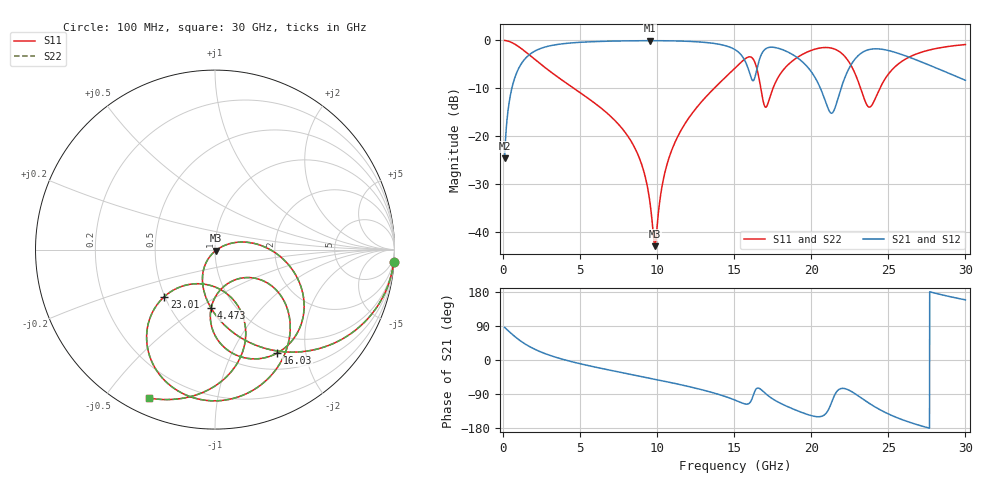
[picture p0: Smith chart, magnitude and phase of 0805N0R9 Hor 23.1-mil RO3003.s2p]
# GHz S MA R 50
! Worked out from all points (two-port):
!   3201 points, 100 MHz to 30 GHz, reference 50 ohm
!   highest |S21| = -0.06 dB at 9.556 GHz (marker M1); lowest = -24.7 dB at 100 MHz (marker M2)
!   |S21| within 3 dB of the highest: 1.679 GHz to 15.46 GHz (13.78 GHz wide, 161 % of centre); 23.09 GHz to 25.96 GHz (2.877 GHz wide, 11.7 % of centre)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
!   lowest |S11| = -43.1 dB at 9.846 GHz (marker M3), VSWR 1.01, Z = 50.4 - j0.57 ohm
!   |S11| at or under -10 dB: 4.578 GHz to 13.71 GHz (9.127 GHz wide, 99.8 % of centre); 16.72 GHz to 17.52 GHz (795.4 MHz wide, 4.65 % of centre); 23.2 GHz to 24.45 GHz (1.256 GHz wide, 5.27 % of centre)
!   |S22| runs from -43.1 to 0.0 dB; largest |S21 - S12| = 0
!   S11 on the Smith chart (normalised r, x): 100 MHz: 1, -30; 4.473 GHz: 0.78, -0.56; 16.03 GHz: 0.72, -1.52; 23.01 GHz: 0.50, -0.31; 30 GHz: 0.07, -0.65
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0.1  0.9983 -3.9  0.05821 86.1  0.05821 86.1  0.9983 -3.9
0.511125  0.9582 -19.3  0.2858 70.7  0.2858 70.7  0.9582 -19.3
1.193219  0.8189 -41.3  0.5729 48.6  0.5729 48.6  0.8189 -41.3
2.594781  0.5394 -70.9  0.8398 18.9  0.8398 18.9  0.5394 -70.9
4.472875  0.3249 -94.0  0.9423 -4.6  0.9423 -4.6  0.3249 -94.0
5.089563  0.2773 -99.9  0.9569 -10.7  0.9569 -10.7  0.2773 -99.9
8.275781  0.08983 -124.2  0.9901 -37.8  0.9901 -37.8  0.08983 -124.2
9.555875  0.01887 -117.4  0.9928 -48.3  0.9928 -48.3  0.01887 -117.4
9.845531  0.007026 -53.6  0.9926 -50.7  0.9926 -50.7  0.007026 -53.6
10.06978  0.01521 8.9  0.9923 -52.5  0.9923 -52.5  0.01521 8.9
11.40594  0.1039 20.7  0.9849 -64.1  0.9849 -64.1  0.1039 20.7
15.05  0.5138 -22.4  0.8002 -105.8  0.8002 -105.8  0.5138 -22.4
16.03109  0.6726 -59.1  0.4368 -111.8  0.4368 -111.8  0.6726 -59.1
16.56369  0.4361 -92.2  0.5759 -74.0  0.5759 -74.0  0.4361 -92.2
17.05891  0.2 -60.6  0.8198 -89.6  0.8198 -89.6  0.2 -60.6
18.43244  0.5438 -41.0  0.7622 -122.5  0.7622 -122.5  0.5438 -41.0
20.03956  0.7903 -70.1  0.46 -147.2  0.46 -147.2  0.7903 -70.1
21.33834  0.8281 -100.6  0.173 -109.7  0.173 -109.7  0.8281 -100.6
23.01087  0.3842 -137.1  0.6846 -93.7  0.6846 -93.7  0.3842 -137.1
23.79575  0.2005 -99.8  0.8047 -115.3  0.8047 -115.3  0.2005 -99.8
25.01978  0.4472 -68.1  0.7824 -142.7  0.7824 -142.7  0.4472 -68.1
30  0.9051 -113.9  0.3825 158.8  0.3825 158.8  0.9051 -113.9
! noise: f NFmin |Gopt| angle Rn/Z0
0.1  0.001476  0.9623  1.359  0.008851
3.417  0.007714  0.7518  19.21  0.006097
6.743  0.01335  0.725  35.79  0.008758
10.06  0.02011  0.7325  51.69  0.01221
13.39  0.03582  0.798  67.04  0.02566
16.7  0.1995  0.952  82.44  0.5284
20.03  0.1952  0.9427  96.57  0.3378
23.35  0.1904  0.9327  110.4  0.2054
26.67  0.1235  0.8858  123.1  0.05388
30  0.1294  0.8803  135.3  0.03468
